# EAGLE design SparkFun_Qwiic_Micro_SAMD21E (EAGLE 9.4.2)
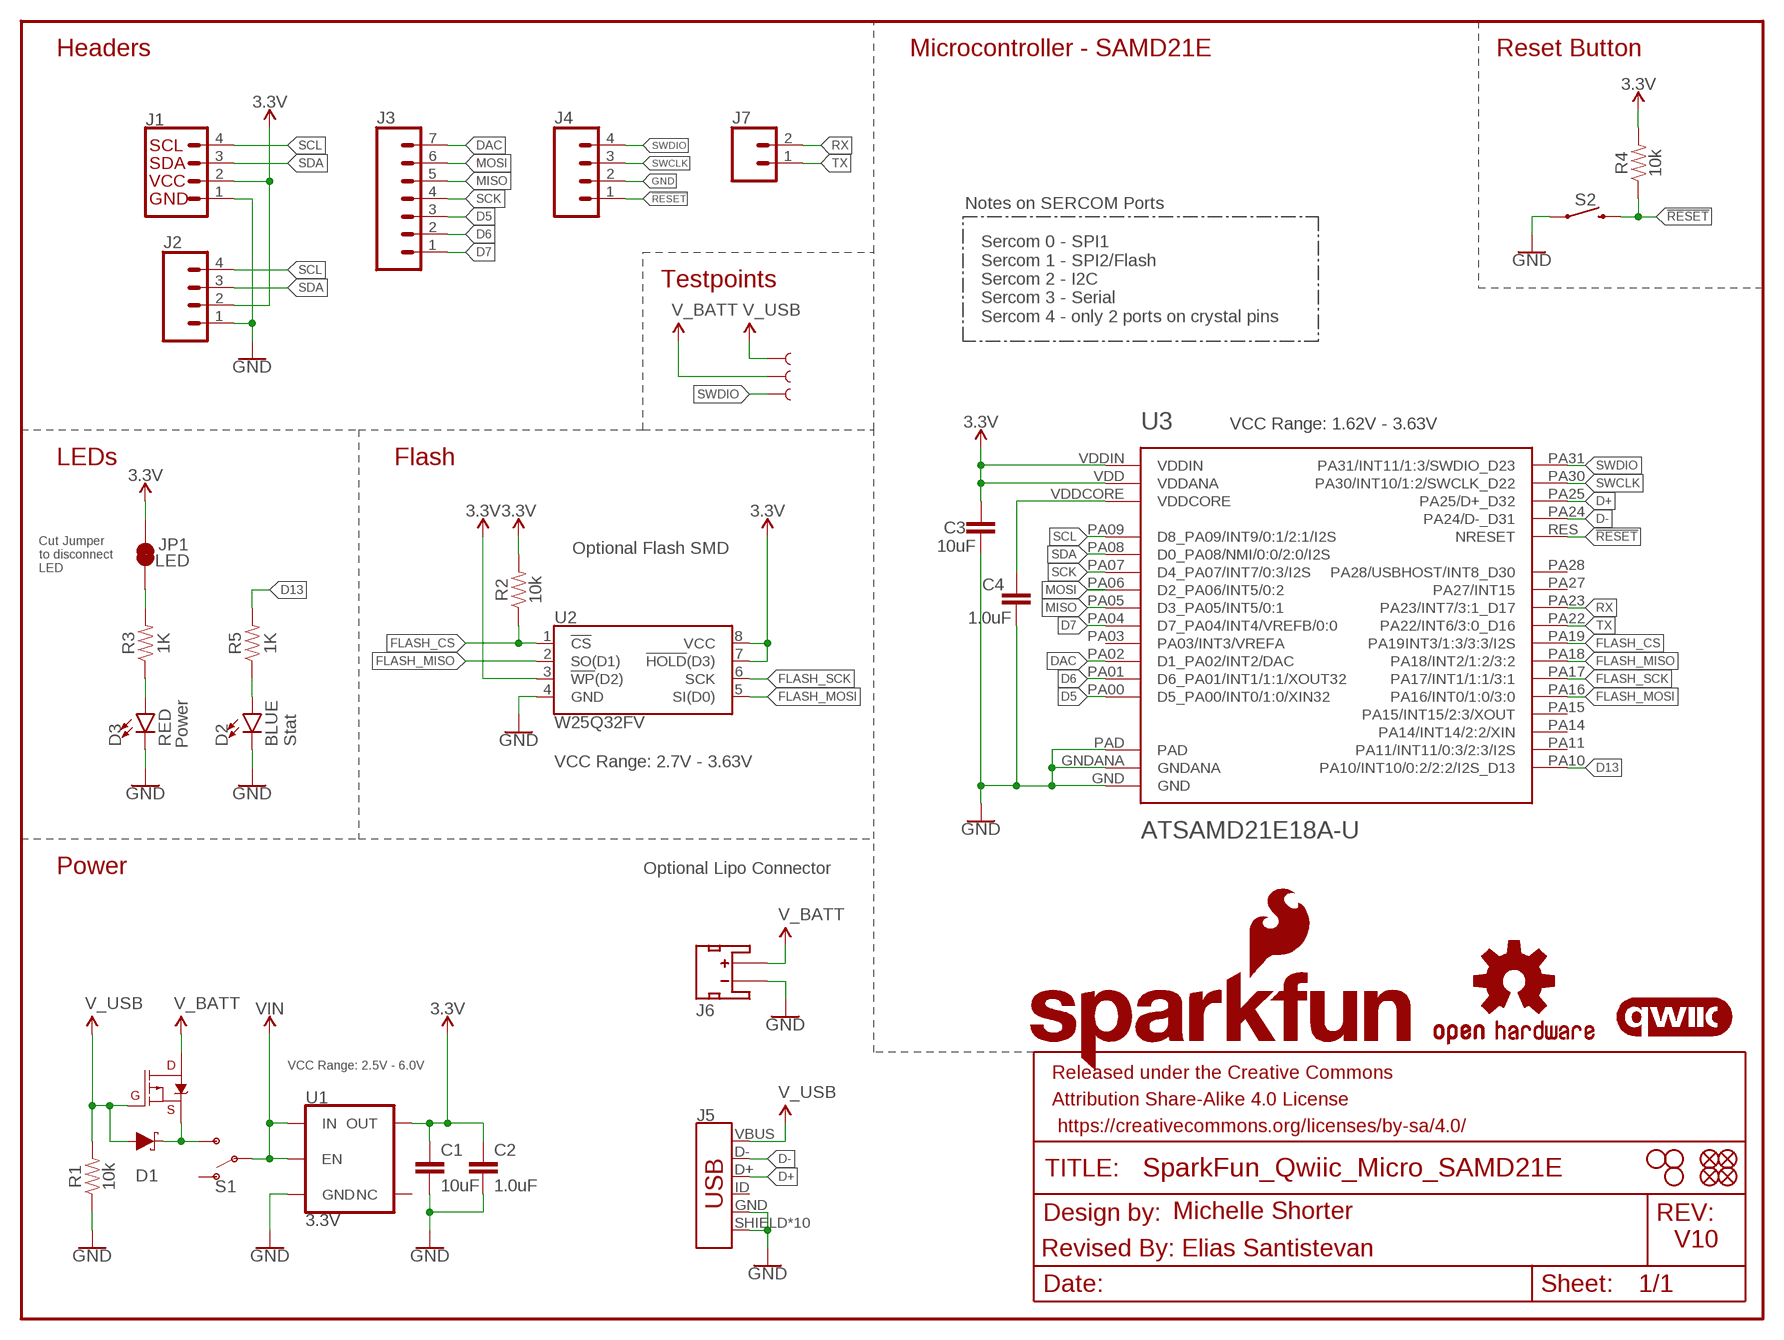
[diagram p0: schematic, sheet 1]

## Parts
C1  10uF  10UF-0603-6.3V-20%  [0603]
C2  1.0uF  1.0UF-0402-16V-10%  [0402]
C3  10uF  10UF-0603-6.3V-20%  [0603]
C4  1.0uF  1.0UF-0402-16V-10%  [0402]
D1  1A/23V/620mV  DIODE-SCHOTTKY-BAT20J  [SOD-323]
D2  BLUE  LED-BLUE0603  [LED-0603]
D3  RED  LED-RED0603  [LED-0603]
FD1  FIDUCIALUFIDUCIAL  [FIDUCIAL-MICRO]
FD2  FIDUCIALUFIDUCIAL  [FIDUCIAL-MICRO]
FD3  FIDUCIALUFIDUCIAL  [FIDUCIAL-MICRO]
FD4  FIDUCIALUFIDUCIAL  [FIDUCIAL-MICRO]
FRAME1  FRAME-LETTER  [CREATIVE_COMMONS]
H1  STAND-OFF  [STAND-OFF]
H2  STAND-OFF  [STAND-OFF]
H3  STAND-OFF  [STAND-OFF]
J1  QWIIC_CONNECTORJS-1MM  [JST04_1MM_RA]
J2  CONN_041X04_NO_SILK  [1X04_NO_SILK]
J3  CONN_07NO_SILK  [1X07_NO_SILK]
J4  CONN_041.27MM_NO_SILK  [1X04_1.27MM_NO_SILK]
J5  USB_MICRO-B_HALF_PTH_MILL  [USB-MICROB-PTH-MILL]
J6  JST_2MM_MALE  [JST-2-SMD]
J7  CONN_021X02_NO_SILK  [1X02_NO_SILK]
JP1  LED  JUMPER-SMT_2_NC_TRACE_SILK  [SMT-JUMPER_2_NC_TRACE_SILK]
LOGO1  SFE_LOGO_NAME.1_INCH  [SFE_LOGO_NAME_.1]
LOGO2  SFE_LOGO_FLAME.2_INCH  [SFE_LOGO_FLAME_.2]
LOGO3  OSHW-LOGOS  [OSHW-LOGO-S]
LOGO4  QWIIC_LOGO_3MM  [QWIIC_3MM]
Q1  3.1A/30V/105mΩ  MOSFET_PCH-DMG2307L  [SOT23-3]
R1  10k  10KOHM-0402-1/16W-1%  [0402]
R2  10k  10KOHM-0402-1/16W-1%  [0402]
R3  1K  1KOHM-0402-1/16W-1%  [0402]
R4  10k  10KOHM-0402-1/16W-1%  [0402]
R5  1K  1KOHM-0402-1/16W-1%  [0402]
S1  SWITCH-SPDT-SMD-RIGHT-ANGLE  [SWITCH_SPST_SMD_A]
S2  MOMENTARY-SWITCH-SPST-SMD-4.6X2.8MM  [TACTILE_SWITCH_SMD_4.6X2.8MM]
TP1  TEST-POINTTP_15TH_THRU  [TP_15TH]
TP2  TEST-POINTTP_15TH_THRU  [TP_15TH]
TP3  TEST-POINTTP_15TH_THRU  [TP_15TH]
U1  3.3V  V_REG_AP2112K-3.3V  [SOT23-5]
U2  W25Q32FV  W25Q32FVSS  [SOIC-8]
U3  ATSAMD21E18A-U  [QFN-32_SAMD]

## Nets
3.3V: C1.1 C2.1 C3.1 J1.2 J2.2 JP1.2 R2.2 R4.2 U1.5(OUT) U2.3(!WP!(D2)) U2.7(!HOLD!(D3)) U2.8(VCC) U3.VDD(VDDANA) U3.VDDIN
!RESET: J4.1 R4.1 S2.3 S2.4 U3.RES(NRESET)
D5: J3.3 U3.PA00(D5_PA00/INT0/1:0/XIN32)
D6: J3.2 U3.PA01(D6_PA01/INT1/1:1/XOUT32)
D7: J3.1 U3.PA04(D7_PA04/INT4/VREFB/0:0)
D13: R5.2 U3.PA10(PA10/INT10/0:2/2:2/I2S_D13)
D+: J5.D+ U3.PA25(PA25/D+_D32)
D-: J5.D- U3.PA24(PA24/D-_D31)
DAC: J3.7 U3.PA02(D1_PA02/INT2/DAC)
FLASH_CS: R2.1 U2.1(!CS!) U3.PA19(PA19INT3/1:3/3:3/I2S)
FLASH_MISO: U2.2(SO(D1)) U3.PA18(PA18/INT2/1:2/3:2)
FLASH_MOSI: U2.5(SI(D0)) U3.PA16(PA16/INT0/1:0/3:0)
FLASH_SCK: U2.6(SCK) U3.PA17(PA17/INT1/1:1/3:1)
GND: C1.2 C2.2 C3.2 C4.1 D2.C D3.C J1.1 J2.1 J4.2 J5.GND J5.SHIELD J5.SHIELD2(SHIELD) J5.SHIELD3(SHIELD) J5.SHIELD4(SHIELD) J5.SHIELD5(SHIELD) J5.SHIELD6(SHIELD) J5.SHIELD7(SHIELD) J5.SHIELD8(SHIELD) J5.SHIELD9(SHIELD) J5.SHIELD10(SHIELD) J6.1(-) R1.1 S2.1 S2.2 U1.2(GND) U2.4(GND) U3.GND U3.GNDANA U3.PAD
MISO: J3.5 U3.PA05(D3_PA05/INT5/0:1)
MOSI: J3.6 U3.PA06(D2_PA06/INT5/0:2)
N$1: D3.A R3.1
N$2: JP1.1 R3.2
N$4: D2.A R5.1
RX: J7.2 U3.PA23(PA23/INT7/3:1_D17)
SCK: J3.4 U3.PA07(D4_PA07/INT7/0:3/I2S)
SCL: J1.4 J2.4 U3.PA09(D8_PA09/INT9/0:1/2:1/I2S)
SDA: J1.3 J2.3 U3.PA08(D0_PA08/NMI/0:0/2:0/I2S)
SWCLK: J4.3 U3.PA30(PA30/INT10/1:2/SWCLK_D22)
SWDIO: J4.4 TP3.P$1 U3.PA31(PA31/INT11/1:3/SWDIO_D23)
TX: J7.1 U3.PA22(PA22/INT6/3:0_D16)
V_BATT: J6.2(+) Q1.3(D) TP2.P$1
V_USB: D1.A J5.VBUS Q1.1(G) R1.2 TP1.P$1
VDDCORE: C4.2 U3.VDDCORE
VIN: S1.2(P) U1.1(IN) U1.3(EN)
VIN1: D1.C Q1.2(S) S1.3(S)
Unconnected: J5.ID J6.NC1(PAD1) J6.NC2(PAD2) S1.1(O) U1.4(NC) U3.PA03(PA03/INT3/VREFA) U3.PA11(PA11/INT11/0:3/2:3/I2S) U3.PA14(PA14/INT14/2:2/XIN) U3.PA15(PA15/INT15/2:3/XOUT) U3.PA27(PA27/INT15) U3.PA28(PA28/USBHOST/INT8_D30)

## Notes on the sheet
- Headers | Microcontroller - SAMD21E | Reset Button
- Notes on SERCOM Ports
- Testpoints
- Sercom 0 - SPI1
  Sercom 1 - SPI2/Flash
  Sercom 2 - I2C
  Sercom 3 - Serial
  Sercom 4 - only 2 ports on crystal pins
- U3 | VCC Range: 1.62V - 3.63V
- LEDs | Flash
- Optional Flash SMD
- Cut Jumper 
  to disconnect
  LED
- Power | Stat
- VCC Range: 2.7V - 3.63V
- Power | Optional Lipo Connector
- VCC Range: 2.5V - 6.0V
- Michelle Shorter
- V10
- Revised By: Elias Santistevan

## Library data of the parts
C1 C3 = SparkFun-Capacitors:10UF: 10.0µF ceramic capacitors; PROD_ID: CAP-11015
C2 C4 = SparkFun-Capacitors:1.0UF: 1µF ceramic capacitors; PROD_ID: CAP-12417
D1 = SparkFun-DiscreteSemi:DIODE-SCHOTTKY: Schottky diode; PROD_ID: DIO-11623
D2 = SparkFun-LED:LED-BLUE: Blue SMD LED; PROD_ID: DIO-08575
D3 = SparkFun-LED:LED-RED: Red SMD LED; PROD_ID: DIO-00819
FD1-FD4 = SparkFun-Aesthetics:FIDUCIAL: Fiducial Alignment Points
FRAME1 = SparkFun-Aesthetics:FRAME-LETTER: Schematic Frame - Letter
H1-H3 = SparkFun-Hardware:STAND-OFF: Stand Off
J1 = SparkFun-Connectors:QWIIC_CONNECTOR: SparkFun I2C Standard Qwiic Connector An SMD 1mm pitch JST connector makes it easy and quick (get it? Qwiic?) to connect I2C devices to each other. The Qwiic system enables fast and solderless connection between popular platforms and various sensors and actuators. We carry 200mm, 100mm, 50mm, and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; PROD_ID: CONN-13694
J2 = SparkFun-Connectors:CONN_04: Multi connection point. Often used as Generic Header-pin footprint for 0.1 inch spaced/style header connections On any of the 0.1 inch spaced packages, you can populate with these: Break Away Headers - Straight (PRT-00116) Break Away Male Headers - Right Angle (PRT-00553) Female Headers (PRT-00115)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; PROD_ID: CONN-09696
J3 = SparkFun-Connectors:CONN_07: Multi connection point. Often used as Generic Header-pin footprint for 0.1 inch spaced/style header connections On any of the 0.1 inch spaced packages, you can populate with these: Break Away Headers - Straight (PRT-00116) Break Away Male Headers - Right Angle (PRT-00553) Female Headers (PRT-00115)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
J4 = SparkFun-Connectors:CONN_04: Multi connection point. Often used as Generic Header-pin footprint for 0.1 inch spaced/style header connections On any of the 0.1 inch spaced packages, you can populate with these: Break Away Headers - Straight (PRT-00116) Break Away Male Headers - Right Angle (PRT-00553) Female Headers (PRT-00115)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
J5 = SparkFun-Connectors:USB_MICRO-B: USB Type Micro-B Connector Male/female and PTH/SMT variants SparkFun Products: SparkFun microB USB Breakout SparkFun USB microB Plug Breakout SparkFun ESP8266 Thing; PROD_ID: CONN-13711
J6 = SparkFun-Connectors:JST_2MM_MALE: JST 2MM MALE RA CONNECTOR Two pin, compact surface mount connector. Commonly used as a battery input connection point. We really like the solid locking feeling and high current rating on these small connectors. We use these all the time as battery connectors. Mates to single-cell LiPo batteries.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; PROD_ID: CONN-11443; SF_ID: PRT-08612
J7 = SparkFun-Connectors:CONN_02: Multi connection point. Often used as Generic Header-pin footprint for 0.1 inch spaced/style header connections
JP1 = SparkFun-Jumpers:JUMPER-SMT_2_NC_TRACE: Normally closed trace jumper
LOGO1 = SparkFun-Aesthetics:SFE_LOGO_NAME: SparkFun Font Logo
LOGO2 = SparkFun-Aesthetics:SFE_LOGO_FLAME: SparkFun Flame Logo
LOGO3 = SparkFun-Aesthetics:OSHW-LOGO: Open-Source Hardware (OSHW) Logo
LOGO4 = SparkFun-Aesthetics:QWIIC_LOGO: Qwiic Logos for placement on schematic and PCB. The 5.5mm silk logo is best for placing next to Qwiic connector.
Q1 = SparkFun-DiscreteSemi:MOSFET_PCH: P-channel MOSFETs Voltage controlled devices that allow control of high current outputs. SparkFun Products: SparkFun ESP32 Thing SparkFun ESP8266 Thing SparkFun Pi Servo HAT V2 DMG2305UX-7 (20V/4.2A/SOT23-3); PROD_ID: TRANS-11308
R1 R2 R4 = SparkFun-Resistors:10KOHM: 10kΩ resistor; PROD_ID: RES-14241
R3 R5 = SparkFun-Resistors:1KOHM: 1kΩ resistor; PROD_ID: RES-14342
S1 = SparkFun-Switches:SWITCH-SPDT: Single Pole, Double Throw (SPDT) Switch Single-pole, double-throw (SPDT) switch. Variant Overview SMD-AYZ0202 Surface Mount DPDT Switch (COM-00597) Used on e.g. LilyPad Arduino USB - ATmega32U4 Board PTH-11.6X4.0MM SPDT Mini Power Switch (COM-00102) Used on e.g. SparkFun Simon Says - Through-Hole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; PROD_ID: SWCH-10651; SF_SKU: COM-10860
S2 = SparkFun-Switches:MOMENTARY-SWITCH-SPST: Momentary Switch (Pushbutton) - SPST; PROD_ID: SWCH-13065
TP1-TP3 = SparkFun-Connectors:TEST-POINT: SparkFun Test Points
U1 = SparkFun-IC-Power:V_REG_AP2112: AP2112 - 600mA CMOS LDO Regulator w/ Enable The AP2112 is CMOS process low dropout linear regulator with enable function, the regulator delivers a guaranteed 600mA (min.) continuous load current. Features Output Voltage Accuracy: ±1.5% Output Current: 600mA (Min.) Foldback Short Current Protection: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; PROD_ID: VREG-12457
U2 = SparkFun-IC-Memory:W25Q32FV: W25Q32FV 32Mb (4MB) Serial Flash Memory The W25Q32FV support the standard Serial Peripheral Interface (SPI), Dual/Quad I/O SPI as well as 2-clocks instruction cycle Quad Peripheral Interface (QPI). 104MHz, SPI, 8-SOIC-EIAJ Datasheet SparkFun Products SparkFun Blynk Board - ESP8266 (WRL-13794); PROD_ID: IC-13229
U3 = SparkFun-IC-Microcontroller:ATSAMD21E18A-U: SAM D21E 32-Pin QFN The SAMD21E is built around the 32-bit ARM Cortex-M0+ processor with up to 256KB of Flash and 32KB of SRAM. It operates at a maximum frequency of 48MHz.; PROD_ID: IC-14428

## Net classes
1 vcc: width 0 mm

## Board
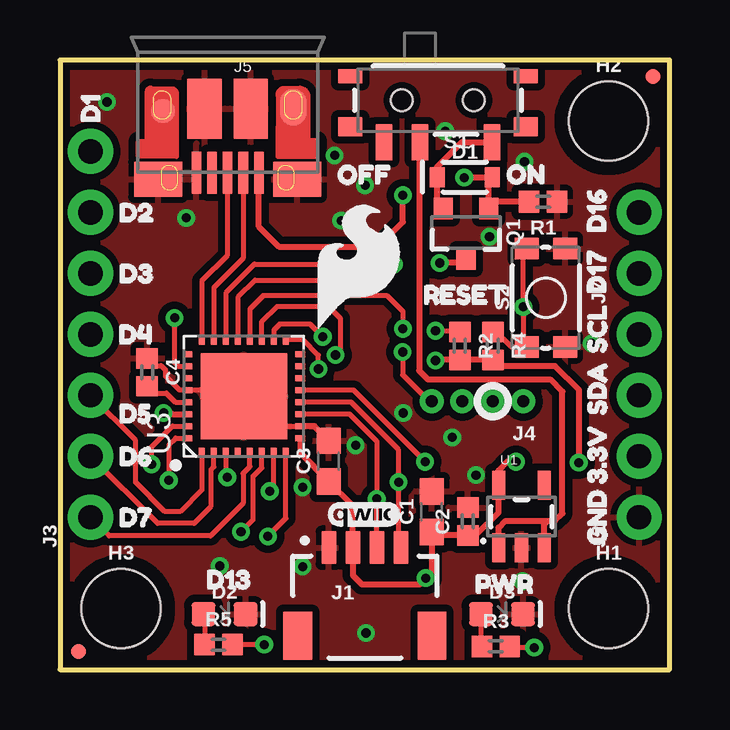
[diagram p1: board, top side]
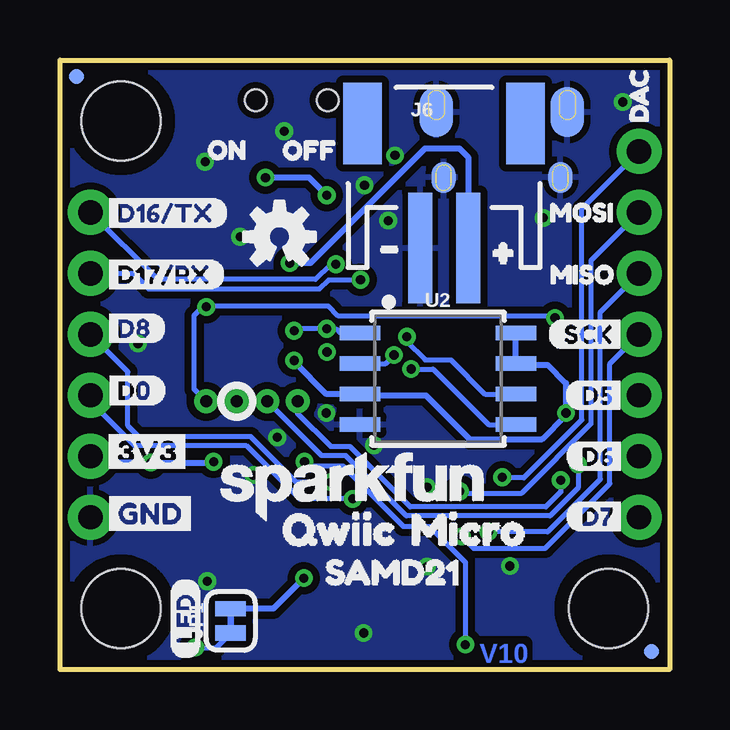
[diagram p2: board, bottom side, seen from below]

Size 25.4 x 25.4 mm. Coordinates in mm from the lower left corner, seen from the top.
Outline: 0,0 25.4,0 25.4,25.4 0,25.4 0,0
Copper layers (1*16): Top 0.035mm / dielectric 1.5mm / Bottom 0.035mm
Design rules "SparkFun-2-layer-TIGHT": minimum track width 7mil, minimum drill 15mil, track to track 7mil, track to pad 7mil, pad to pad 7mil, via to via 7mil, smd to smd 7mil, copper to edge 7mil, drill to drill 7mil, minimum pad ring 7mil, minimum via ring 7mil, stop-mask expansion 4mil, vias tented up to drill 25mil, thermal gap 10mil

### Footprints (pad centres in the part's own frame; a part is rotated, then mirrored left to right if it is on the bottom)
0603 = smd 1.1 x 1: 1 -0.85,0; 2 0.85,0
0402 = smd 0.85 x 0.9: 1 -0.58,0; 2 0.58,0
SOD-323 = smd 0.63 x 0.83: A 1.15,0; C -1.15,0
LED-0603 = smd 1 x 1: A -0.877,0; C 0.877,0
FIDUCIAL-MICRO = smd 0.635 x 0.635: 1 0,0
STAND-OFF = hole 3.302: 0,0
JST04_1MM_RA = smd 0.6 x 1.35: 1 -1.5,0; 2 -0.5,0; 3 0.5,0; 4 1.5,0 | smd 1.2 x 2: NC1 2.8,-3.675; NC2 -2.8,-3.675
1X04_NO_SILK = drill 1.016 pad 1.88: 1 0,0; 2 2.54,0; 3 5.08,0; 4 7.62,0
1X07_NO_SILK = drill 1.016 pad 1.88: 1 0,0; 2 2.54,0; 3 5.08,0; 4 7.62,0; 5 10.16,0; 6 12.7,0; 7 15.24,0
1X04_1.27MM_NO_SILK = drill 0.508 pad 1: 1 0,0; 2 1.27,0; 3 2.54,0; 4 3.81,0
USB-MICROB-PTH-MILL = smd 0.4 x 1.75: D+ 0,0; D- -0.65,0; GND 1.3,0; ID 0.65,0; VBUS -1.3,0 | smd 2 x 1.46: SHIELD -2.9,0.275; SHIELD2 2.9,0.275 | smd 1.425 x 2.5: SHIELD3 -0.963,-2.675; SHIELD4 0.963,-2.675 | smd 1.4 x 2.1 bottom: SHIELD5 -2.731,-2.531; SHIELD7 2.729,-2.531 | smd 1 x 1: SHIELD6 2.7,-2.575 | smd 1.1 x 1.5: SHIELD8 -2.731,-2.731 | smd 1 x 1.3 bottom: SHIELD9 -2.43,0.195; SHIELD10 2.43,0.195
JST-2-SMD = smd 1 x 4.6: 1 -1,-3.7; 2 1,-3.7 | smd 1.6 x 3.4: NC1 -3.4,1.5; NC2 3.4,1.5
1X02_NO_SILK = drill 1.016 pad 1.88: 1 0,0; 2 2.54,0
SMT-JUMPER_2_NC_TRACE_SILK = smd 0.635 x 1.27: 1 -0.508,0; 2 0.508,0
SOT23-3 = smd 0.8 x 0.9: 1 -0.95,-1; 2 0.95,-1; 3 0,1.1
SWITCH_SPST_SMD_A = smd 0.7 x 1.5: 1 -2.25,-1.75; 2 -0.75,-1.75; 3 2.25,-1.75 | smd 1 x 0.6: GND1 -3.65,1; GND3 3.65,1 | smd 1 x 0.8: GND2 -3.65,-1.1; GND4 3.65,-1.1 | hole 0.9: -1.5,0; 1.5,0
TACTILE_SWITCH_SMD_4.6X2.8MM = smd 0.9 x 1: 1 -2.05,-0.8; 2 2.05,-0.8; 3 2.05,0.8; 4 -2.05,0.8
TP_15TH = drill 0.381 pad 0.61: P$1 0,0
SOT23-5 = smd 0.55 x 1.2: 1 -0.95,-1.3; 2 0,-1.3; 3 0.95,-1.3; 4 0.95,1.3; 5 -0.95,1.3
SOIC-8 = smd 0.61 x 1.702: 1 -1.905,-3.251; 2 -0.635,-3.251; 3 0.635,-3.251; 4 1.905,-3.251; 5 1.905,3.251; 6 0.635,3.251; 7 -0.635,3.251; 8 -1.905,3.251
QFN-32_SAMD = smd 0.25 x 0.4: GND 0.21,2.31; GNDANA -1.29,-2.39; PA08 -0.79,-2.39; PA09 -0.29,-2.39; PA10 0.21,-2.39; PA11 0.71,-2.39; PA14 1.21,-2.39; PA15 1.71,-2.39; PA27 1.71,2.31; PA28 0.71,2.31; PA30 -1.29,2.31; PA31 -1.79,2.31; RES 1.21,2.31; VDD -1.79,-2.39; VDDCORE -0.29,2.31; VDDIN -0.79,2.31 | smd 0.4 x 0.25: PA00 -2.39,1.71; PA01 -2.39,1.21; PA02 -2.39,0.71; PA03 -2.39,0.21; PA04 -2.39,-0.29; PA05 -2.39,-0.79; PA06 -2.39,-1.29; PA07 -2.39,-1.79; PA16 2.31,-1.79; PA17 2.31,-1.29; PA18 2.31,-0.79; PA19 2.31,-0.29; PA22 2.31,0.21; PA23 2.31,0.71; PA24 2.31,1.21; PA25 2.31,1.71 | smd 3.6 x 3.6: PAD -0.04,-0.04

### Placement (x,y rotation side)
C1  15.49,6.58 90 top
C2  16.99,6.17 90 top
C3  11.2,8.69 90 top
C4  3.63,12.39 270 top
D1  16.87,20.52 0 top
D2  6.86,2.31 0 top
D3  18.41,2.31 0 top
FD1  24.71,24.71 0 bottom
FD2  0.76,0.76 0 top
FD3  24.71,24.71 0 top
FD4  0.76,0.76 0 bottom
FRAME1  not placed on the board
H1  22.86,2.54 0 top
H2  22.86,22.86 0 top
H3  2.54,2.54 0 top
J1  12.7,5.08 0 top
J2  24.13,6.35 90 top
J3  1.27,6.35 90 top
J4  19.3,11.18 180 top
J5  6.99,20.7 180 top
J6  9.4,21.26 0 bottom
J7  24.13,16.51 90 top
JP1  18.29,2.03 90 bottom
LOGO1  13.21,7.62 0 bottom
LOGO2  12.45,16.76 0 top
LOGO3  16.26,18.03 0 bottom
LOGO4  12.66,6.46 0 top
Q1  16.92,18.21 180 top
R1  20.13,19.49 180 top
R2  16.66,13.49 270 top
R3  18.16,0.97 0 top
R4  18.03,13.49 270 top
R5  6.6,1.04 0 top
S1  15.75,23.72 0 top
S2  20.24,15.49 90 top
TP1  16.84,20.5 0 top
TP2  15.82,16.94 0 top
TP3  14.27,13.23 0 top
U1  19.23,6.38 0 top
U2  9.65,12.12 270 bottom
U3  7.62,11.43 90 top
U$1  [D00]  23.72,11.63 0 bottom
U$2  [GND-03]  23.77,6.5 0 bottom
U$3  [#23]  13.21,17.78 0 bottom
U$4  [#24]  8.51,17.53 0 bottom
U$5  [3#3V10]  22.38,7.06 90 top
U$6  [D12]  1.27,22.1 90 top
U$7  [D166]  22.35,17.53 90 top
U$8  [D177]  22.35,14.99 90 top
U$9  [D16#TX4]  23.7,19.02 0 bottom
U$10  [QWIIC2]  17.27,5.84 0 bottom
U$11  [D17#RX3]  23.7,16.46 0 bottom
U$12  [D75]  1.78,6.35 0 top
U$13  [DAC1]  1.27,22.1 90 bottom
U$14  [MISO0]  5.68,16.46 0 bottom
U$15  [SAMD213]  15.24,4.06 0 bottom
U$16  [MOSI2]  5.69,19.05 0 bottom
U$17  [3V3-03]  23.83,9.09 0 bottom
U$18  [ON12]  19.93,21.65 0 bottom
U$19  [OFF13]  16.8,21.64 0 bottom
U$20  [SCK7]  5.23,13.97 0 bottom
U$21  [RESET0]  14.45,15.62 0 top
U$22  [D85]  23.7,14.22 0 bottom
U$23  [MICRO2]  11.94,5.84 0 bottom
U$24  [LED1]  20.17,0.39 90 bottom
U$25  [D50]  4.37,11.43 0 bottom
U$26  [D61]  4.37,8.89 0 bottom
U$27  [D72]  4.37,6.38 0 bottom
U$28  [D21]  1.78,19.05 0 top
U$29  [D136]  5.41,3.76 0 top
U$36  [D33]  1.78,16.51 0 top
U$37  [D41]  1.78,13.97 0 top
U$38  [D52]  1.79,10.67 0 top
U$39  [D65]  1.78,8.89 0 top
U$44  [GND11]  22.38,4.52 90 top
U$45  [OFF13]  10.88,20.62 0 top
U$46  [ON12]  17.92,20.64 0 top
U$47  [PWR16]  16.64,3.57 0 top
U$49  [SCL8]  22.38,12.52 90 top
U$50  [SDA9]  22.38,9.93 90 top

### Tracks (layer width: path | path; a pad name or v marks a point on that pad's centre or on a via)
3.3V  (via drill 0.38)
  Top 0.254: v4.32,10.69 4.62,10.69 4.67,10.64 U3.VDDIN | v19,8.66 18.64,8.66 18.28,8.3 U1.5 18.28,6.54 17.33,5.59 C2.1 15.63,5.59 C1.1 15.49,4.06 v15.24,3.81 14.99,3.56 12.57,3.56 12.2,3.93 J1.2 12.2,6.84 C3.1 10.01,9.03 U3.VDD | v21.61,8.62 21.61,11.66 20.62,12.65 18.29,12.65 R4.2 R2.2 15.68,12.91 v15.65,12.88
  Bottom 0.203: U2.7 6.35,12.7 6.02,12.7
  Bottom 0.254: v19,8.66 19.04,8.62 v21.61,8.62 23.1,8.62 23.37,8.89 J2.2 | U2.7 U2.8 | 6.02,12.7 5.08,12.7 4.32,11.94 v4.32,10.69 4.32,10.59 5.31,9.6 8.33,9.6 10.16,11.43 12.85,11.43 U2.3 14.3,11.48 15.65,12.83 v15.65,12.88 | v15.24,3.81 16.51,2.54 JP1.2
!RESET  (via drill 0.38)
  Top 0.203: v4.78,14.66 4.78,12.78 4.91,12.64 U3.RES | R4.1 18.31,13.79 18.46,13.79 18.81,13.44 S2.4 19.3,13.58 v19.3,15.11 19.3,17.4 S2.3
  Bottom 0.203: J4.1 19.81,11.68 19.81,14.76 19.46,15.11 v19.3,15.11 19.27,15.15 14.22,15.15 13.8,14.73 4.85,14.73 v4.78,14.66
D5
  Top 0.203: U3.PA00 5.91,7.49 5,6.58 4.37,6.58 3.15,7.8 3.15,9.55 J3.3
D6
  Top 0.203: J3.2 4.06,6.1 5.59,6.1 6.3,6.81 6.3,8.33 6.41,8.44 U3.PA01
D7
  Top 0.203: U3.PA04 7.91,8.46 7.63,8.18 7.63,6.93 6.27,5.58 2.04,5.58 J3.1
D13  (via drill 0.38)
  Top 0.203: v15.21,8.66 12.24,11.64 U3.PA10 | v8.51,1.04 R5.2
  Bottom 0.203: v8.51,1.04 8.51,4.47 10.01,5.97 11.1,5.97 13.61,8.48 15.04,8.48 v15.21,8.66
D+
  Top 0.203: U3.PA25 5.91,16.2 6.99,17.27 J5.D+
D-
  Top 0.203: J5.D- 7.63,17.14 6.41,15.92 U3.PA24
DAC  (via drill 0.38)
  Top 0.203: U3.PA02 6.91,8.08 v6.97,8.01
  Bottom 0.203: v6.97,8.01 6.95,7.99 6.07,7.99 3.66,10.4 3.66,19.2 J3.7
FLASH_CS  (via drill 0.38)
  Top 0.203: v14.29,14.2 14.29,14.92 13.61,15.6 8.48,15.6 7.91,15.02 U3.PA19 | v15.65,14.12 16.61,14.12 R2.1
  Bottom 0.203: U2.1 13.72,14.02 13.89,14.2 v14.29,14.2 15.57,14.2 v15.65,14.12
FLASH_MISO  (via drill 0.38)
  Top 0.203: v11.48,13.11 11.68,13.31 11.68,14.63 11.18,15.14 9.04,15.14 8.41,14.51 U3.PA18
  Bottom 0.203: U2.2 11.84,12.75 v11.48,13.11
FLASH_MOSI  (via drill 0.38)
  Top 0.203: v10.77,12.52 10.77,13.11 10.14,13.74 U3.PA16
  Bottom 0.203: v10.77,12.52 9.86,12.52 7.54,10.21 U2.5
FLASH_SCK  (via drill 0.38)
  Top 0.203: v10.95,13.87 10.41,14.4 9.17,14.4 8.91,14.14 U3.PA17
  Bottom 0.203: v10.95,13.87 10.95,13.66 10.19,12.9 9.12,12.9 7.7,11.48 U2.6
GND  (via drill 0.38)
  Top 0.203: 3.92,12.67 4.21,12.67 4.39,12.49 4.39,12.23 4.98,11.64 U3.GND 6.1,11.64 6.35,11.39 U3.PAD 8.15,11.39 9.4,10.14 U3.GNDANA
  Top 0.254: C4.1 3.92,12.67 | C3.2 10.6,10.14 U3.GNDANA
  other vias: 19.27,3.68 5.26,18.82 11.72,18.71 14.3,10.69 19.35,21.16 22.15,13.59 10.11,7.59 12.75,1.52 17.89,18.03 10.11,4.29 12.32,9.35 6.65,4.32 1.96,23.65 17.34,8.1 16.34,9.68 16.05,22.43 11.44,21.42 12.71,20.18
  pour Top (isolate 0.305): 0,0 0,25.4 25.4,25.4 25.4,0
  pour Bottom (isolate 0.305): 0,25.4 25.4,25.4 25.4,0 0,0
MISO  (via drill 0.38)
  Top 0.203: v7.54,5.74 8.04,6.24 8.04,8.04 8.41,8.41 U3.PA05
  Bottom 0.203: J3.5 2.88,14.9 2.88,7.94 5.08,5.74 v7.54,5.74
MOSI  (via drill 0.38)
  Top 0.203: v8.74,7.43 8.91,7.6 U3.PA06
  Bottom 0.203: v8.74,7.43 8.66,7.35 6.16,7.35 3.28,10.24 3.28,17.04 J3.6
N$1
  Top 0.203: D3.A 17.54,1.01 R3.1
N$2  (via drill 0.38)
  Top 0.203: v19.76,0.91 18.79,0.91 R3.2
  Bottom 0.203: v19.76,0.91 18.9,0.91 JP1.1
N$4
  Top 0.203: D2.A 6.02,2.27 R5.1
RX  (via drill 0.38)
  Top 0.203: v13.91,16.89 8.1,16.89 6.91,15.7 U3.PA23
  Bottom 0.203: v13.91,16.89 14.12,16.89 14.76,16.26 21.34,16.26 J7.2
SCK  (via drill 0.38)
  Top 0.203: v8.66,5.55 9.41,6.3 U3.PA07
  Bottom 0.203: v8.66,5.55 8.17,5.05 5.18,5.05 2.49,7.75 2.49,12.75 J3.4
SCL  (via drill 0.38)
  Top 0.203: U3.PA09 12.13,11.14 14.11,9.16 v14.11,7.81 14.11,5.17 J1.4
  Bottom 0.203: J2.4 22.57,12.41 22.57,10.16 22.11,9.7 17.45,9.7 15.56,7.81 v14.11,7.81
SDA  (via drill 0.38)
  Top 0.203: J1.3 v13.2,7.11 13.2,9.51 12.07,10.64 U3.PA08
  Bottom 0.203: J2.3 24.13,11.18 22.28,9.32 17.63,9.32 15.42,7.11 v13.2,7.11
SWCLK  (via drill 0.38)
  Top 0.203: v3.81,8.56 3.81,9.27 4.68,10.14 U3.PA30
  Bottom 0.203: v3.81,8.56 3.81,7.57 4.98,6.4 10.97,6.4 13.49,8.91 14.5,8.91 J4.3
SWDIO  (via drill 0.38)
  Top 0.203: v4.53,7.89 4.53,9.36 4.81,9.64 U3.PA31 | TP3.P$1 14.28,12.28 15.38,11.18 J4.4
  Bottom 0.203: v4.53,7.89 4.53,7.4 5.16,6.78 10.81,6.78 13.32,9.3 14.12,9.3 15.49,10.67 J4.4
TX  (via drill 0.38)
  Top 0.203: v12.88,16.24 12.87,16.23 8.13,16.23 7.41,15.51 U3.PA22
  Bottom 0.203: J7.1 22.35,16.51 21.7,15.86 14.59,15.86 14.21,16.24 v12.88,16.24
V_BATT
  Top 0.254: Q1.3 16.75,16.94 TP2.P$1
  Bottom 0.254: TP2.P$1 14.96,16.94 10.19,21.72 8.76,21.72 8.4,21.35 J6.2
V_USB  (via drill 0.38)
  Top 0.254: R1.2 18.15,19.49 Q1.1 17.87,20.37 D1.A 17.99,20.5 TP1.P$1 | J5.VBUS 8.29,18.46 9.12,17.63 13.26,17.63 14.29,18.66 v14.29,19.76
  Bottom 0.254: v14.29,19.76 15.02,20.5 TP1.P$1
VDDCORE
  Top 0.203: 3.92,11.52 4.43,11.52 4.81,11.14 U3.VDDCORE
  Top 0.254: C4.2 3.92,11.52
VIN
  Top 0.254: S1.2 14.96,21.94 14.96,12.46 15.33,12.09 20.42,12.09 20.93,11.58 20.93,6.5 20.62,6.2 20.32,6.2 | U1.1 18.28,5.92 18.56,6.2 20.32,6.2 | U1.3 20.18,6.05 20.32,6.2
VIN1
  Top 0.254: Q1.2 15.72,19.46 D1.C 15.72,20.95 16.74,21.97 S1.3

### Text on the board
Bottom: V10
Measures: Units in Inches
tDocu: Michelle Shorter | Revised By: Elias Santistevan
